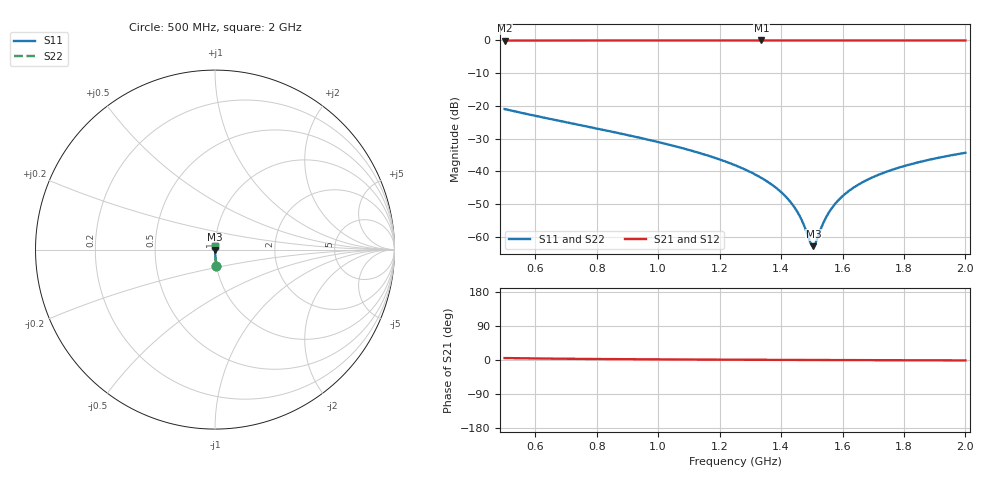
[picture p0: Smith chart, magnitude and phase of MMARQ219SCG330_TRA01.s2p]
! MMARQ219SCG330_TRA01  S-PARAMETER MODEL  ( General Type )
! Model Generated by TAIYO YUDEN Corporation (http://www.ty-top.com)
! Version 1.0
! TAIYO YUDEN Control No. 150609
! Copyright(c) 2015 TAIYO YUDEN CO.,LTD. All Rights Reserved.
! Product Description (link to TY-COMPAS)
! https://ds.yuden.co.jp/TYCOMPAS/or/detail?pn=MMARQ219SCG330JTRA01&u=M
! Products Name : Multilayer Ceramic Capacitors
! Characteristics :
!  Capacitance : 33 pF , Rated Voltage : 250V , TCC : CG / C0G
!  Case Size : 2.0 x 1.25 / 0.079 x 0.049 [mm/inch] , Thickness : 0.85 / 0.033 [mm/inch]
!  (Conditions: Temperature = 25 degC , DC Bias Current/Voltage = 0A / 0V)
! External Node Assignments :
!  1  o---| |---o  2
! GND o---------o GND
! Frequency Range : 500MHz  -  2GHz  [ 401 STEP ]
# MHz S RI R 50
! Freq[MHz].  S11 Real  S11 Imag  S21 Real  S21 Imag  S12 Real  S12 Imag  S22 Real  S22 Imag
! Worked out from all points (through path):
!   401 points, 500 MHz to 2 GHz, reference 50 ohm
!   highest |S21| = -0.01 dB at 1.336 GHz (marker M1); lowest = 0.0 dB at 500 MHz (marker M2)
!   group delay of S21, straight-line fit = 10.2 ps
!   lowest |S11| = -62.8 dB at 1.505 GHz (marker M3), VSWR 1.00, Z = 50.1 + j0.00364 ohm
!   |S11| at or under -10 dB: start of sweep to end of sweep
!   |S22| runs from -62.8 to -20.9 dB; largest |S21 - S12| = 0
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500  0.00835 -0.0893  0.9917 0.0893  0.9917 0.0893  0.00835 -0.0893
751.25  0.00294 -0.0503  0.9971 0.0503  0.9971 0.0503  0.00294 -0.0503
1002.5  0.0013 -0.0279  0.9987 0.0279  0.9987 0.0279  0.0013 -0.0279
1141.25  0.00093 -0.0187  0.9991 0.0187  0.9991 0.0187  0.00093 -0.0187
1250  0.000781 -0.0125  0.9992 0.0125  0.9992 0.0125  0.000781 -0.0125
1336.25  0.000723 -0.00794  0.9993 0.00794  0.9993 0.00794  0.000723 -0.00794
1392.5  0.000709 -0.00516  0.9993 0.00516  0.9993 0.00516  0.000709 -0.00516
1433.75  0.000708 -0.00321  0.9993 0.00321  0.9993 0.00321  0.000708 -0.00321
1463.75  0.000712 -0.00182  0.9993 0.00182  0.9993 0.00182  0.000712 -0.00182
1493.75  0.00072 -0.000465  0.9993 0.000465  0.9993 0.000465  0.00072 -0.000465
1501.25  0.000723 -0.00013  0.9993 0.00013  0.9993 0.00013  0.000723 -0.00013
1505  0.000724 3.64e-05  0.9993 -3.64e-05  0.9993 -3.64e-05  0.000724 3.64e-05
1512.5  0.000727 0.000369  0.9993 -0.000369  0.9993 -0.000369  0.000727 0.000369
1535  0.000737 0.00136  0.9993 -0.00136  0.9993 -0.00136  0.000737 0.00136
1553.75  0.000746 0.00217  0.9993 -0.00217  0.9993 -0.00217  0.000746 0.00217
1572.5  0.000757 0.00297  0.9992 -0.00297  0.9992 -0.00297  0.000757 0.00297
1595  0.000771 0.00392  0.9992 -0.00392  0.9992 -0.00392  0.000771 0.00392
1625  0.000793 0.00516  0.9992 -0.00516  0.9992 -0.00516  0.000793 0.00516
1662.5  0.000824 0.00669  0.9992 -0.00669  0.9992 -0.00669  0.000824 0.00669
1752.5  0.000913 0.0102  0.9991 -0.0102  0.9991 -0.0102  0.000913 0.0102
1865  0.00105 0.0145  0.9989 -0.0145  0.9989 -0.0145  0.00105 0.0145
2000  0.00125 0.0192  0.9987 -0.0192  0.9987 -0.0192  0.00125 0.0192
